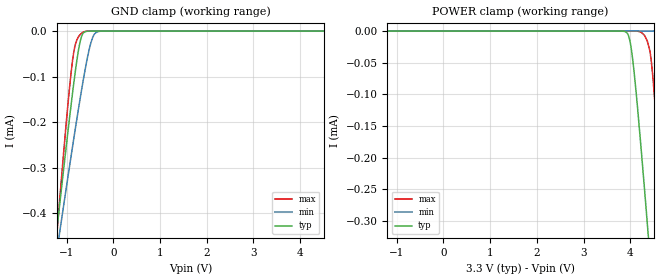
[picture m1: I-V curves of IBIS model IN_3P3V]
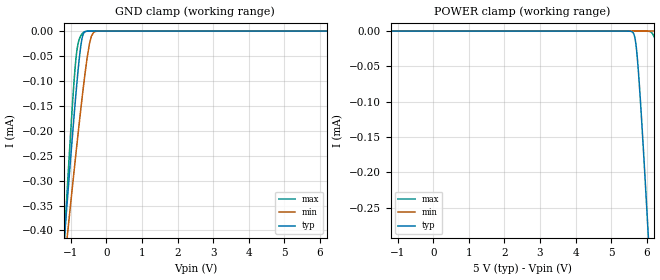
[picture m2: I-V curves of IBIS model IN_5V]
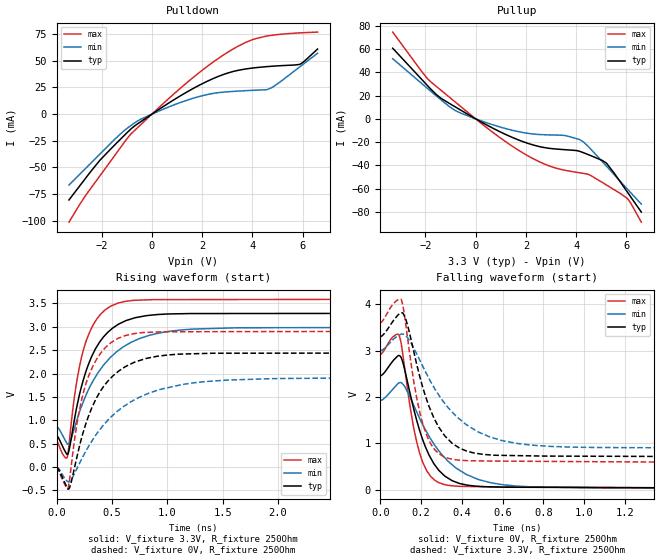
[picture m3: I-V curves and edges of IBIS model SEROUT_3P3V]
| Texas Instruments Incorporated
| Automotive Power Logic 8-Bit Shift Register LED Driver
| Marketing part#   Voltage Range   Package-type   #pins/pkg drawing
| TLC6C598DRQ1   3.0V - 5.5V   SOIC   16/D
| TLC6C598PWRQ1   3.0V - 5.5V   TSSOP   16/PW
[IBIS Ver]   4.1
[File name]   tlc6c598.ibs
[File Rev]   1.0
[Date]   11/19/2013
[Source]   Model built from spectre simulations at:
   Texas Instruments Incorporated.
   Analog-eLab, HPA
   12500 TI Blvd
   Dallas, TX -75243
   For Support e-mail: elab_ibis@list.ti.com
[Notes]   Revision History
   Rev 1.0: 11/19/2013
   - ccomp values are based on PVT settings:
   MIN: Low Voltage, High Temperature, Weak Process
   TYP: Nominal Voltage, Nominal Temperature, Nominal Process
   MAX: High Voltage, Low Temperature, Fast Process
   - C_comp although listed in numerical order of value are obtained from varying PVT conditions.
   For PVT conditions for each specific value, refer to the buffer description under respective [Model].
   IBIS model user is responsible for using appropriate C_comp to simulate for Signal Integrity.
[Disclaimer]  This model is designed as an aid for customers of Texas Instruments
 TI and its licensors and suppliers make no warranties, either expressed
 or implied, with respect to this  model, including the warranties of
 merchantability or fitness for a particular purpose.
 The model is provided solely on an "as is" basis. The entire risk as to
 its quality and performance is with the customer.
[Copyright] (C)Copyright 2013 Texas Instruments Incorporated.
   All rights reserved.
[Component]   TLC6D598D
[Manufacturer]  Texas Instruments Incorporated
[Package]   |16-pin SOIC D package
|   typ   min   max
R_pkg   0.0606   0.0545   0.0702
L_pkg   1.8889n   1.6309n   2.1736n
C_pkg   0.1987p   0.1601p   0.2295p
[Pin]   signal_name   model_name   R_pin   L_pin   C_pin
1   VCC   POWER   0.0610   1.9985n  0.2290p
2   SERIN   IN   0.0591   1.8353n  0.2097p
3   DRAIN0   DRAIN   0.0649   1.9780n  0.1894p
4   DRAIN0   DRAIN   0.0548   1.6350n  0.1604p
5   DRAIN0   DRAIN   0.0545   1.6351n  0.1604p
6   DRAIN0   DRAIN   0.0702   2.1736n  0.2005p
7   CLRB   IN   0.0590   1.8459n  0.2107p
8   GB   IN   0.0609   2.0154n  0.2294p
9   SEROUT   SEROUT   0.0608   2.0072n  0.2295p
10   RCK   IN   0.0591   1.8553n  0.2101p
11   DRAIN0   DRAIN   0.0649   1.9851n  0.1898p
12   DRAIN0   DRAIN   0.0549   1.6352n  0.1604p
13   DRAIN0   DRAIN   0.0548   1.6309n  0.1601p
14   DRAIN0   DRAIN   0.0702   2.1589n  0.2001p
15   SRCK   IN   0.0594   1.8372n  0.2103p
16   GND   GND   0.0616   1.9956n  0.2290p
[Component]   TLC6D598PW
[Manufacturer]  Texas Instruments Incorporated
[Package]   |16-pin TSSOP PW package
|   typ   min   max
R_pkg   0.1251   0.0788   0.1363
L_pkg   2.7951n   2.4754n   3.3005n
C_pkg   0.4710p   0.4062p   0.5687p
[Pin]   signal_name   model_name   R_pin   L_pin   C_pin
1   VCC   POWER   0.0796   2.8517n  0.5687p
2   SERIN   IN   0.1357   2.9894n  0.5314p
3   DRAIN0   DRAIN   0.1338   2.6345n  0.4099p
4   DRAIN0   DRAIN   0.1246   2.4848n  0.4065p
5   DRAIN0   DRAIN   0.1248   2.4876n  0.4065p
6   DRAIN0   DRAIN   0.1344   2.6436n  0.4090p
7   CLRB   IN   0.1356   2.9828n  0.5277p
8   GB   IN   0.1305   3.2476n  0.5155p
9   SEROUT   SEROUT   0.1341   3.3005n  0.5150p
10   RCK   IN   0.1360   2.9819n  0.5246p
11   DRAIN0   DRAIN   0.1344   2.6349n  0.4083p
12   DRAIN0   DRAIN   0.1248   2.4782n  0.4062p
13   DRAIN0   DRAIN   0.1246   2.4754n  0.4062p
14   DRAIN0   DRAIN   0.1338   2.6257n  0.4096p
15   SRCK   IN   0.1363   2.9918n  0.5325p
16   GND   GND   0.0788   2.9105n  0.5586p
[Model Selector] IN
IN_5V   IN 5.0V INPUT
IN_3P3V   IN 3.3V INPUT
[Model Selector] SEROUT
SEROUT_5V   SEROUT 5.0V OUTPUT
SEROUT_3P3V   SEROUT 3.3V OUTPUT
[Model Selector] DRAIN
DRAIN_5V   DRAIN 5.0V OPEN-DRAIN OUTPUT
DRAIN_3P3V   DRAIN 3.3V OPEN-DRAIN OUTPUT
| Models and submodels in the file (6): IN_3P3V (Input), IN_5V (Input), SEROUT_3P3V (Output), SEROUT_5V (Output), DRAIN_3P3V (Open_drain), DRAIN_5V (Open_drain)
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|   Model IN_3P3V
[Model]   IN_3P3V
Model_type   Input
Vinl = .7
Vinh = 2.4
|   typ   min   max
|   (nom PVT)   (slow PVT)   (fast PVT)
C_comp   2.39f   2.18f   2.52f
[Voltage Range]   3.3   3   3.6
[Temperature Range]   27   150   -40
[Power Clamp Reference]   3.3   3   3.6
[GND Clamp Reference]   -0   -0   -0
[GND Clamp]
|   Voltage   I(typ)   I(min)   I(max)
-3.3V     -2.421mA   -1.967mA   -3.113mA
-1.251V   -478.3uA   -514.6uA   -499.8uA
-1.181V   -413.6uA   -466.2uA   -413.1uA
-1.162V   -395.2uA   -452.4uA   -388.5uA
-983.4mV  -232.8uA   -329.5uA   -175.7uA
-864.6mV  -130.4uA   -249.3uA   -59.27uA
-805.2mV  -83.47uA   -210.1uA   -27.08uA
-735.9mV  -36.91uA   -165.4uA   -11.32uA
-636.9mV  -3.805uA   -104.6uA   -2.006uA
-438.9mV  -9.03nA    -13.51uA   -3.643nA
-270.6mV  0A         -219.5nA   0A
6.59V     0A         0A         0A
[POWER Clamp]
|   Voltage   I(typ)   I(min)   I(max)
-3.3V     0A         0A         0A
3.887V    -858.9nA   0A         -776.5pA
3.967V    -8.744uA   0A         -1.062nA
4.026V    -31.48uA   0A         -3.554nA
4.105V    -83.47uA   0A         -50.11nA
4.224V    -180.6uA   0A         -1.491uA
4.363V    -304.1uA   0A         -15.93uA
4.412V    -349.5uA   0A         -29.63uA
4.452V    -386uA     0A         -50.23uA
4.521V    -450.5uA   0A         -109.1uA
4.719V    -637.1uA   0A         -336.1uA
6.59V     -2.412mA   0A         -2.727mA
|   Model IN_5V
[Model]   IN_5V
Model_type   Input
Vinl = .7
Vinh = 2.4
|   typ   min   max
|   (nom PVT)   (slow PVT)   (fast PVT)
C_comp   2.39f   2.18f   2.52f
[Voltage Range]   5   4.5   5.5
[Temperature Range]   27   150   -40
[Power Clamp Reference]   5   4.5   5.5
[GND Clamp Reference]   -0   -0   -0
[GND Clamp]
|   Voltage   I(typ)   I(min)   I(max)
-5V       -3.931mA   -3.128mA   -5.089mA
-1.25V    -477.7uA   -514.1uA   -498.9uA
-1.13V    -366uA     -430.5uA   -349.5uA
-1.04V    -283.6uA   -368.3uA   -241uA
-920mV    -177.5uA   -286.6uA   -108.1uA
-845mV    -114.5uA   -236.3uA   -45.97uA
-725mV    -30.95uA   -158.5uA   -9.749uA
-665mV    -8.38uA    -121.3uA   -3.614uA
-605mV    -1.461uA   -86.23uA   -931.5nA
-425mV    -5.121nA   -10.37uA   -1.338nA
-275mV    0A         -247nA     0A
9.985V    0A         0A         0A
[POWER Clamp]
|   Voltage   I(typ)   I(min)   I(max)
-5V       0A         0A         0A
5.605V    -1.464uA   0A         -1nA
5.68V     -12.28uA   0A         -1.051nA
5.74V     -39.28uA   0A         -1.11nA
5.845V    -114.5uA   0A         -1.323nA
6.04V     -283.6uA   0A         -151.3nA
6.085V    -324.6uA   0A         -551.9nA
6.235V    -463.6uA   0A         -11.19uA
6.325V    -548.2uA   0A         -35.15uA
6.4V      -619.1uA   0A         -88.97uA
6.58V     -790.2uA   0A         -288.7uA
9.985V    -3.918mA   0A         -4.52mA
|   Model SEROUT_3P3V
[Model]   SEROUT_3P3V
Model_type   Output
Polarity   Inverting
Vmeas = 1.65
Vref = 3.3
Cref = 0pF
Rref = 250
|   typ   min   max
|   (nom PVT)   (slow PVT)   (fast PVT)
C_comp   1.514p   1.378p   1.654p
|C_comp (ON state)   1.627p   1.606p   1.677p
|C_comp (OFF state)   1.514p   1.378p   1.654p
[Voltage Range]   3.3   3   3.6
[Temperature Range]   27   150   -40
[Pullup Reference]   3.3   3   3.6
[Pulldown Reference]   -0   -0   -0
[Power Clamp Reference]   3.3   3   3.6
[GND Clamp Reference]   -0   -0   -0
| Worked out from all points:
|   slope of the pulldown table from 0 to 0.495 V, typ, clamps not added: 63.8 ohm
|   slope of the pullup table from 0 to 0.495 V, typ, clamps not added: 83.8 ohm
|   falling waveform, V_fixture 0V, R_fixture 250Ohm: 20-80 % time 121ps typ, 204ps min, 79.7ps max; typ from 2.46 V to 0.011 V
|   rising waveform, V_fixture 3.3V, R_fixture 250Ohm: 20-80 % time 244ps typ, 376ps min, 176ps max; typ from 0.675 V to 3.29 V
|   rising waveform, V_fixture 0V, R_fixture 250Ohm: 20-80 % time 300ps typ, 509ps min, 205ps max; typ from 0 V to 2.44 V
|   falling waveform, V_fixture 3.3V, R_fixture 250Ohm: 20-80 % time 134ps typ, 240ps min, 85.3ps max; typ from 3.3 V to 0.685 V
[Pulldown]
|   Voltage   I(typ)   I(min)   I(max)
-3.3V     -80.58mA   -66.54mA   -101.5mA
-2.637V   -60.12mA   -50.96mA   -76.34mA
-2.062V   -43.13mA   -37.33mA   -57.76mA
-933.9mV  -16.15mA   -12.39mA   -21.34mA
-607.2mV  -9.751mA   -6.986mA   -13.51mA
838.2mV   12.92mA    8.296mA    18.21mA
2.095V    29.63mA    17.8mA     42.9mA
3.472V    41.29mA    21.68mA    64.28mA
4.58V     44.6mA     23.02mA    73.33mA
5.026V    45.33mA    28.98mA    74.75mA
5.877V    46.71mA    44.26mA    76.26mA
6.59V     61.07mA    57.16mA    77.01mA
[Pullup]
|   Voltage   I(typ)   I(min)   I(max)
-3.3V     60.68mA    51.66mA    74.54mA
-1.924V   28.72mA    26.25mA    34.67mA
-1.379V   17.66mA    16.29mA    24.55mA
-825mV    10.43mA    7.3mA      14.69mA
699.6mV   -8.223mA   -5.22mA    -11.91mA
2.561V    -23.96mA   -13.51mA   -37.17mA
3.521V    -26.47mA   -14.27mA   -44.06mA
4.155V    -28.05mA   -18.06mA   -46.43mA
4.541V    -31.29mA   -25.18mA   -48.28mA
5.194V    -37.92mA   -40.47mA   -56.72mA
6.036V    -62.94mA   -60.35mA   -68.56mA
6.59V     -80.13mA   -73.26mA   -88.82mA
[Ramp]
R_load = 250
|   typ   min   max
dV/dt_r   1.56945/2.4352e-10   1.27665/3.75911e-10   1.82362/1.75703e-10
dV/dt_f   1.46589/1.20841e-10   1.14378/2.03708e-10   1.74488/7.97528e-11
[Falling Waveform]
V_fixture = 0V
V_fixture_min = 0V
V_fixture_max = 0V
R_fixture = 250Ohm
C_fixture = 0F
|   Time   V(typ)   V(min)   V(max)
0s        2.455V     1.921V     2.916V
91.94ps   2.896V     2.303V     3.332V
111.2ps   2.739V     2.274V     2.902V
156.4ps   1.884V     1.893V     1.517V
193.5ps   1.272V     1.534V     780.6mV
247.2ps   681.9mV    1.092V     282.6mV
333.1ps   244.5mV    608.7mV    90.89mV
480.1ps   69.96mV    218.1mV    61.63mV
743.6ps   47.86mV    56.9mV     54.36mV
4.9ns     11.38mV    14.63mV    7.482mV
[Rising Waveform]
V_fixture = 3.3V
V_fixture_min = 3V
V_fixture_max = 3.6V
R_fixture = 250Ohm
C_fixture = 0F
|   Time   V(typ)   V(min)   V(max)
0s        675.4mV    864.9mV    554.8mV
94.43ps   269.2mV    499.8mV    194mV
115.1ps   379.1mV    512.1mV    529.6mV
178.5ps   1.235V     961.4mV    1.77V
266.6ps   2.052V     1.542V     2.69V
396.6ps   2.697V     2.09V      3.268V
555.2ps   3.05V      2.489V     3.508V
834.3ps   3.245V     2.816V     3.579V
1.234ns   3.284V     2.952V     3.583V
4.9ns     3.291V     2.993V     3.594V
[Rising Waveform]
V_fixture = 0V
V_fixture_min = 0V
V_fixture_max = 0V
R_fixture = 250Ohm
C_fixture = 0F
|   Time   V(typ)   V(min)   V(max)
0s        652.3pV    132.4nV    452.3pV
103ps     -472.2mV   -320.3mV   -459.1mV
127.7ps   -368.7mV   -284.1mV   -80.89mV
193.5ps   307.2mV    10.66mV    1.05V
286ps     1.071V     424.9mV    1.925V
438.7ps   1.765V     935.9mV    2.551V
619.5ps   2.144V     1.316V     2.812V
934.3ps   2.377V     1.659V     2.891V
1.534ns   2.435V     1.859V     2.897V
4.9ns     2.444V     1.911V     2.909V
[Falling Waveform]
|Gnd
V_fixture = 3.3V
V_fixture_min = 3V
V_fixture_max = 3.6V
R_fixture = 250Ohm
C_fixture = 0F
|   Time   V(typ)   V(min)   V(max)
0s        3.3V       3V         3.6V
103ps     3.818V     3.357V     4.1V
127.7ps   3.643V     3.311V     3.48V
166ps     2.949V     3.04V      2.292V
208.5ps   2.207V     2.662V     1.42V
266.6ps   1.516V     2.181V     864.1mV
361.8ps   972.1mV    1.632V     646.4mV
539.4ps   746.9mV    1.132V     614.9mV
834.3ps   721.6mV    931.3mV    606.8mV
4.9ns     685.2mV    878.4mV    561mV
